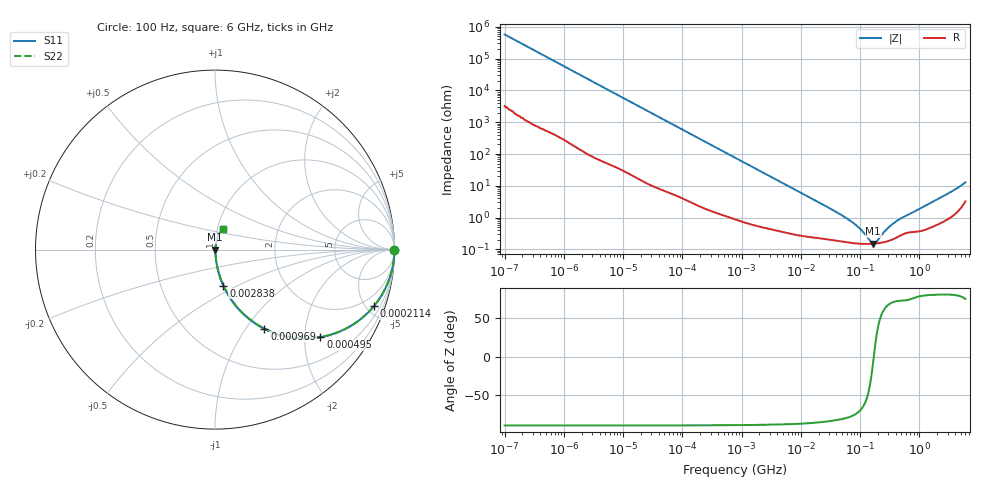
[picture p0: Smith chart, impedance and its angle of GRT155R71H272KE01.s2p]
!Murata Part Number: GRT155R71H272KE01
!These Parameters are Measured in Series Mode Connection
!Data Generated on Jun 19, 2026
!  o--ll--o
!Port1  Port2
!  o------o
!Operation Temp=25[degC], DC Bias Voltage=0[V]
!Freq. Start=100[Hz] Stop=6[GHz] 401[Steps]
# Hz S RI R 50
!Freq.(Hz) S11(Real) S11(Imag) S21(Real) S21(Imag) S12(Real) S12(Imag) S22(Real) S22(Imag)
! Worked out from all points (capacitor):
!   401 points, 100 Hz to 6 GHz, reference 50 ohm
!   read as one part in series: C = 2.76 nF near 109 Hz
!   lowest |Z| = 151 mohm at 166.9 MHz (marker M1)
!   series resonance near 170.6 MHz, so ESL is about 320 pH
!   S11 on the Smith chart (normalised r, x): 100 Hz: open; 211.4 kHz: 1.04, -5.58; 495 kHz: 1.02, -2.39; 969 kHz: 1.02, -1.23; 2.838 MHz: 1.01, -0.42; 6 GHz: 1.06, +0.25
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100  1 -0.000174  1e-06 0.000174  1e-06 0.000174  1 -0.000174
2008  1 -0.00346  2.7e-05 0.00346  2.7e-05 0.00346  1 -0.00346
40335  0.9949 -0.0685  0.0051 0.0685  0.0051 0.0685  0.9949 -0.0685
94437  0.9738 -0.1563  0.0262 0.1563  0.0262 0.1563  0.9738 -0.1563
211427  0.8842 -0.3162  0.1158 0.3162  0.1158 0.3162  0.8842 -0.3162
316350  0.775 -0.4134  0.225 0.4134  0.225 0.4134  0.775 -0.4134
495019  0.5874 -0.4874  0.4126 0.4874  0.4126 0.4874  0.5874 -0.4874
774597  0.371 -0.4774  0.629 0.4774  0.629 0.4774  0.371 -0.4774
968953  0.2756 -0.4406  0.7244 0.4406  0.7244 0.4406  0.2756 -0.4406
1585629  0.1274 -0.3258  0.8726 0.3258  0.8726 0.3258  0.1274 -0.3258
2837864  0.0464 -0.2  0.9536 0.2  0.9536 0.2  0.0464 -0.2
6075234  0.0128 -0.0975  0.9872 0.0975  0.9872 0.0975  0.0128 -0.0975
1.555665e7  0.00388 -0.0386  0.9961 0.0386  0.9961 0.0386  0.00388 -0.0386
7.129496e7  0.00164 -0.00733  0.9984 0.00733  0.9984 0.00733  0.00164 -0.00733
1.020051e8  0.00151 -0.00401  0.9985 0.00401  0.9985 0.00401  0.00151 -0.00401
1.526266e8  0.00149 -0.000834  0.9985 0.000834  0.9985 0.000834  0.00149 -0.000834
1.669249e8  0.0015 -0.00016  0.9985 0.00016  0.9985 0.00016  0.0015 -0.00016
1.909225e8  0.00154 0.000849  0.9985 -0.000849  0.9985 -0.000849  0.00154 0.000849
3.124326e8  0.00189 0.00479  0.9981 -0.00479  0.9981 -0.00479  0.00189 0.00479
4.888888e8  0.00283 0.00898  0.9972 -0.00898  0.9972 -0.00898  0.00283 0.00898
2.34314e9  0.00858 0.0423  0.9914 -0.0423  0.9914 -0.0423  0.00858 0.0423
6e9  0.0451 0.1145  0.9549 -0.1145  0.9549 -0.1145  0.0451 0.1145
